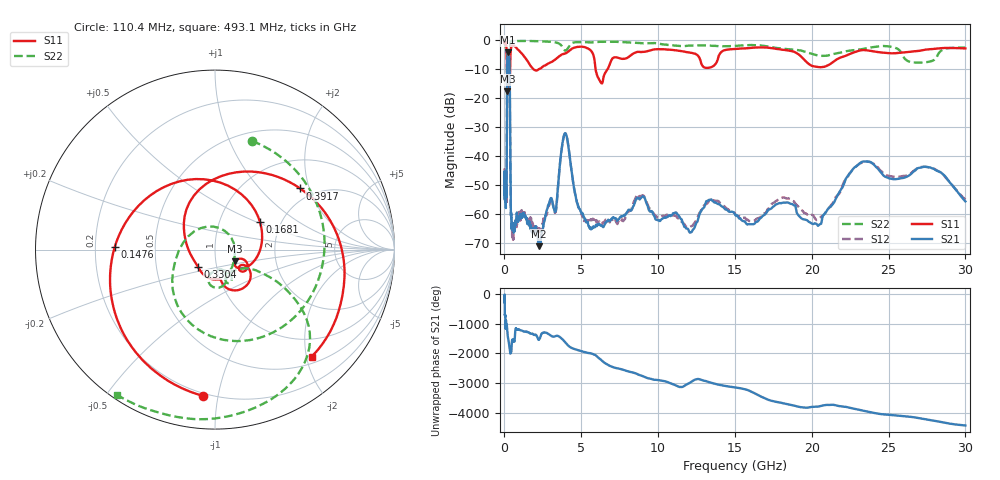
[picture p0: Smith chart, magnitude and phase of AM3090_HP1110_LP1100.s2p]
! Date/Time: Thu, Feb 28, 2019 2:09 PM
! Network Analyzer: Agilent Technologies E8364B Rev: A.07.50.67
! Sweep from 0.010 to 30.000 GHz, 1601 Points, Sweep Type: LOG
! Power Supply: 5.022 V, 0.002 A
# Hz S DB R 50
!freq MagS11 AngS11 MagS21 AngS21 MagS12 AngS12 MagS22 AngS22
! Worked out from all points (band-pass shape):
!   1601 points, 10 MHz to 30 GHz, reference 50 ohm
!   highest |S21| = -4.16 dB at 243.5 MHz (marker M1); lowest = -71.2 dB at 2.246 GHz (marker M2)
!   |S21| within 3 dB of the highest: 177.3 MHz to 325 MHz (147.6 MHz wide, 58.8 % of centre)
!   lowest |S11| = -17.8 dB at 193.4 MHz (marker M3), VSWR 1.30, Z = 62 - j8.2 ohm
!   |S11| at or under -10 dB: 166.1 MHz to 361.1 MHz (195 MHz wide, 74 % of centre); 1.867 GHz to 2.256 GHz (389 MHz wide, 18.9 % of centre); 5.93 GHz to 6.719 GHz (788.9 MHz wide, 12.5 % of centre)
!   |S22| runs from -19.2 to -0.1 dB; largest |S21 - S12| = 0.0098
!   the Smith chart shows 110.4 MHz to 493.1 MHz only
!   S11 on the Smith chart (normalised r, x): 110.4 MHz: 0.18, -0.90; 147.6 MHz: 0.28, +0.01; 168.1 MHz: 1.56, +0.53; 330.4 MHz: 0.81, -0.16; 391.7 MHz: 1.68, +1.74; 493.1 MHz: 0.62, -2.10
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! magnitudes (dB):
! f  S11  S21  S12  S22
! 10 MHz  -0.3  -49.2  -48.4  -0.6
! 38.04 MHz  -0.3  -51.0  -50.4  -1.3
! 110.4 MHz  -1.8  -52.6  -54.5  -3.9
! 144.7 MHz  -4.5  -47.9  -48.9  -5.0
! 147.6 MHz  -5.1  -44.5  -44.3  -5.3
! 168.1 MHz  -10.6  -11.6  -11.6  -18.6
! 193.4 MHz  -17.8  -5.1  -5.1  -16.2
! 243.5 MHz  -15.3  -4.2  -4.1  -18.4
! 330.4 MHz  -17.4  -8.0  -8.0  -10.4
! 391.7 MHz  -4.7  -50.2  -51.0  -0.8
! 493.1 MHz  -1.9  -64.1  -65.4  -0.2
! 550.5 MHz  -1.9  -64.3  -68.9  -0.2
! 2.084 GHz  -10.5  -65.6  -66.0  -0.4
! 2.246 GHz  -10.0  -71.2  -65.2  -0.4
! 3.318 GHz  -6.7  -59.3  -59.5  -0.8
! 3.934 GHz  -4.7  -32.2  -32.3  -3.6
! 5.446 GHz  -2.9  -63.6  -62.5  -0.8
! 6.234 GHz  -14.3  -63.8  -63.1  -0.6
! 7.926 GHz  -6.3  -59.9  -60.4  -0.8
! 20 GHz  -8.9  -63.4  -60.4  -4.8
! 23.48 GHz  -3.5  -42.0  -42.1  -2.9
! 30 GHz  -2.9  -55.8  -55.1  -2.6
